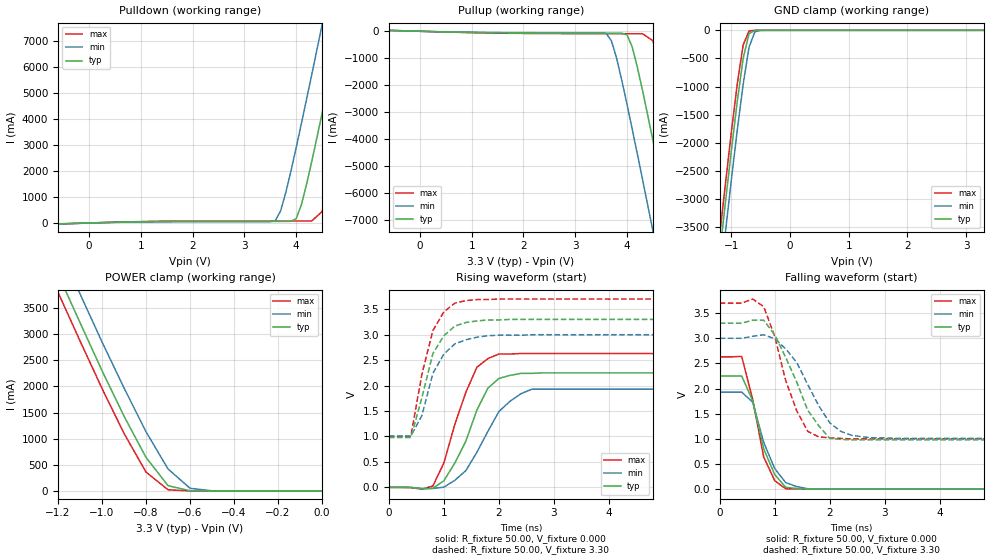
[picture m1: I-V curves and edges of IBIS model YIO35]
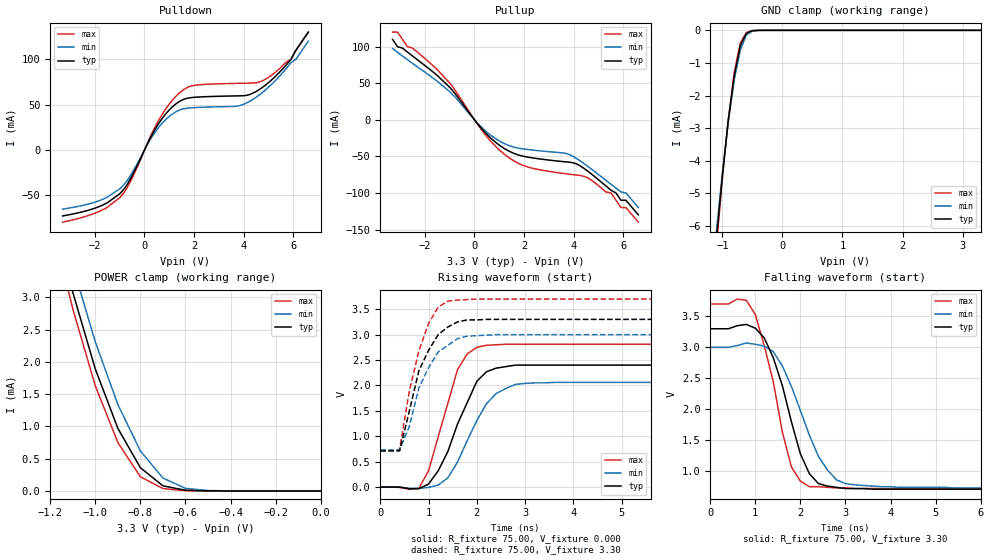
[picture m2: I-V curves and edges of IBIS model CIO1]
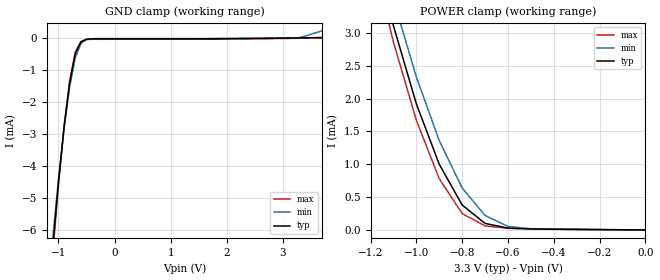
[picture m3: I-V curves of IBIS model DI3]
|   * 9e4101a.ibs * IBIS 2.1 Model file
| Components:
| ICS9e4101a   CK410 CLOCK
| Rev History
| Rev No.   Description
| 1.0   Initial release with Updated Parasitic Parameters
[IBIS Ver]   2.1
[Comment char]  |_char
[File name]   9e4101a.ibs
[Date]   Jan. 27, 2004
[File Rev]   1.0
[Source]   Originated at Integrated Circuit Systems, Inc.
[Disclaimer] (C) Copyright Integrated Circuit Systems, Inc. 2002
   All rights reserved
ICS hereby grants the user of this IBIS model a non-exclusive,
nontransferable license to use this IBIS model under the following terms.
Before using this IBIS model, the user should read this license.
If the user does not accept these terms,  the IBIS model should be
returned to ICS within 30 days.
   The user is granted this license only to use the IBIS model and
is not granted rights to sell, load, rent, lease or license the IBIS
model in whole or in part, or in modified form to anyone other than
user. User may modify the IBIS model to suit its specific
applications but rights to derivative works and such modifications
shall belong to ICS.
   This IBIS model is provided on an "AS IS" basis and ICS makes
absolutely no warranty with respect to the information contained
herein. ICS DISCLAIMS AND CUSTOMER WAIVES ALL WARRANTIES, EXPRESS
OR IMPLIED, INCLUDING WARRANTIES OF MERCHANTABILITY OR FITNESS FOR
A PARTICULAR PURPOSE. The entire risk as to quality and performance
is with the Customer. ACCORDINGLY, IN NO EVENT SHALL THE COMPANY BE
LIABLE FOR ANY DAMAGES, WHETHER IN CONTRACT OR TORT,INCLUDING ANY
LOST PROFITS OR OTHER INCIDENTAL, CONSEQUENTIAL, EXEMPLARY, OR
PUNITIVE DAMAGES ARISING OUT OF THE USE OR APPLICATION OF THE IBIS
model provided in this package. Further, ICS reserves the right to
make changes without notice to any product herein to improve
reliability, function, or design. ICS does not convey any license
under patent rights or any other intellectual property rights,
including those of third parties.
   ICS is not obligated to provide maintenance or support
for the licensed IBIS model.
|   COMPONENT: ICS9e4101a
[Component]   ICS9e4101a
[Manufacturer]  ICS
[Package]
| variable   typ   min   max
R_pkg   81.1m   62.2m   100.0m
L_pkg   6.7nH   4.9nH   8.5nH
C_pkg   0.53pF  0.21pF  0.85pF
[Pin]   signal_name   model_name   R_pin   L_pin   C_pin
  1   VDDPCI   POWER
  2   GND   GND
  3   PCI_3   YO49
  4   PCI_4   YO49
  5   PCI_5   YO49
  6   GND   GND
  7   VDDPCI   POWER
  8   PCI_F0/ITP_EN   YIO35
  9   PCI_F1   YO49
 10   PCI_F2   YO49
 11   VDD48   POWER
 12   USB48   YO49
 13   GND   GND
 14   DOT_96   YH15
 15   DOT_96#   YH15
 16   FS_B   YI5
 17   VTT_PWRGD#   YI3
 18   FS_A   YI5
 19   SRC_1   YH16
 20   SRC_1#   YH16
 21   VDDSRC   POWER
 22   SRC_2   YH16
 23   SRC_2#   YH16
 24   SRC_3   YH16
 25   SRC_3#   YH16
 26   SRC_4_SATA   YH16
 27   SRC_4_SATA#   YH16
 28   VDDSRC   POWER
 29   GND   GND
 30   SRC_5#   YH16
 31   SRC_5   YH16
 32   SRC_6#   YH16
 33   SRC_6   YH16
 34   VDDSRC   POWER
 35   CPU_2_ITP#/SRC_7#   YH17
 36   CPU_2_ITP/SRC_7   YH17
 37   VDD_A   POWER
 38   GND   GND
 39   IREF   YI4
 40   CPU_1#   YH17
 41   CPU_1   YH17
 42   VDDCPU   POWER
 43   CPU_0#   YH17
 44   CPU_0   YH17
 45   GND   GND
 46   SCL   DI3
 47   SDA   DIOSDA
 48   VDDREF   POWER
 49   XTAL_OUT   DIX
 50   XTAL_IN   DIX
 51   GND   GND
 52   REF   YO39
 53   FS_C   YI5
 54   PCI_0   YO49
 55   PCI_1   YO49
 56   PCI_2   YO49
|* Either 3.3V or 2.5V
|** All model are simulated with typical corner process
[Diff Pin]   inv_pin   vdiff   tdelay_typ
14   15   NA   NA
19   20   NA   NA
22   23   NA   NA
24   25   NA   NA
26   27   NA   NA
31   30   NA   NA
33   32   NA   NA
36   35   NA   NA
41   40   NA   NA
44   43   NA   NA
| Models and submodels in the file (15): YIO35 (I/O), CIO1 (I/O), DI3 (Input), DIOSDA (I/O_open_drain), DIX (Input), YI3 (Input), YI4 (Input), YI5 (Input), YH15 (Open_source), YH16 (Open_source), YH17 (Open_source), YO32 (Open_source), YO49 (Output), YO34 (Output), YO39 (Output)
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|   Model YIO35
[Model]   YIO35
Model_type   I/O
Polarity   Non-Inverting
Enable   Active-High
Vinl =   0.80V
Vinh =   2.00V
C_comp   5.50pF   5.00pF   6.00pF
[Temperature Range]   27.00   70.00   0.000
[Voltage Range]   3.30V   3.00V   3.70V
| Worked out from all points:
|   slope of the pulldown table from 0 to 0.495 V, typ, clamps not added: 18 ohm
|   slope of the pullup table from 0 to 0.495 V, typ, clamps not added: 20.5 ohm
|   GND clamp passes 1 mA (typ) near -0.55 V on its own axis
|   POWER clamp passes 1 mA (typ) near -0.53 V on its own axis
|   rising waveform, R_fixture 50.00, V_fixture 0.000: 20-80 % time 547ps typ, 623ps min, 483ps max; typ from 0 V to 2.25 V
|   rising waveform, R_fixture 50.00, V_fixture 3.30: 20-80 % time 399ps typ, 392ps min, 356ps max; typ from 0.98 V to 3.3 V
|   falling waveform, R_fixture 50.00, V_fixture 0.000: 20-80 % time 354ps typ, 371ps min, 324ps max; typ from 2.25 V to 0 V
|   falling waveform, R_fixture 50.00, V_fixture 3.30: 20-80 % time 577ps typ, 609ps min, 450ps max; typ from 3.3 V to 0.98 V
[Pulldown]
| voltage   I(typ)   I(min)   I(max)
|  -3.30   0.000A   0.000A   0.000A
|  -3.10   0.000A   0.000A   0.000A
|  -2.90   0.000A   0.000A   0.000A
|  -2.70   0.000A   0.000A   0.000A
|  -2.50   -10.00mA   0.000A   0.000A
|  -2.30   0.000A   0.000A   0.000A
|  -2.10   -10.00mA   0.000A   0.000A
|  -1.90   0.000A   -10.00mA   0.000A
|  -1.70   -1.00mA   -1.00mA   -1.00mA
|  -1.50   -1.00mA   -1.00mA   -2.00mA
|  -1.00   -4.00mA   -4.00mA   -5.00mA
|  -0.90   -7.00mA   -5.00mA   -9.40mA
|  -0.80   -14.40mA   -8.40mA   -22.50mA
|  -0.70   -32.67mA   -17.10mA   -41.37mA
-600mV    -35.01mA   -28.6mA    -38.03mA
3.6V      62.06mA    99.79mA    76.5mA
3.7V      62.12mA    470mA      76.56mA
4V        170mA      2.9A       76.74mA
4.1V      700mA      3.82A      76.82mA
4.3V      2.36A      5.7A       77.36mA
4.5V      4.21A      7.62A      440mA
4.7V      6.12A      9.55A      2.04A
4.9V      8.05A      11.49A     3.88A
5.1V      9.99A      13.45A     5.79A
5.3V      11.94A     15.41A     7.72A
6.6V      24.78A     28.25A     20.51A
[Pullup]
| voltage   I(typ)   I(min)   I(max)
|  -3.30   0.000A   0.000A   0.000A
|  -3.10   0.000A   0.000A   0.000A
|  -2.90   0.000A   0.000A   0.000A
|  -2.70   0.000A   0.000A   0.000A
|  -2.50   0.000A   0.000A   0.000A
|  -2.30   0.000A   0.000A   0.000A
|  -2.10   10.00mA   0.000A   0.000A
|  -1.90   0.000A   0.000A   0.000A
|  -1.70   1.00mA   1.00mA   1.00mA
|  -1.50   2.00mA   1.00mA   1.00mA
|  -1.00   4.00mA   3.00mA   5.00mA
|  -0.90   6.00mA   4.00mA   8.00mA
|  -0.80   11.80mA   7.00mA   18.80mA
|  -0.70   27.70mA   13.70mA   39.15mA
-600mV    32.94mA    25.47mA    36.47mA
3.6V      -71.61mA   -83.61mA   -90.07mA
3.8V      -72.17mA   -1.01A     -90.7mA
4V        -130mA     -2.71A     -91.27mA
4.1V      -580mA     -3.63A     -91.54mA
4.3V      -2.2A      -5.5A      -92.39mA
4.5V      -4.04A     -7.41A     -350mA
4.7V      -5.94A     -9.34A     -1.9A
4.9V      -7.87A     -11.28A    -3.73A
5.1V      -9.81A     -13.24A    -5.63A
5.3V      -11.76A    -15.2A     -7.56A
6.6V      -24.57A    -28.02A    -20.33A
[GND_clamp]
| voltage   I(typ)   I(min)   I(max)
-3.3V     -24.49A    -24.99A    -24.19A
-1.2V     -3.97A     -4.5A      -3.64A
-1.1V     -3.04A     -3.57A     -2.71A
-1V       -2.13A     -2.65A     -1.8A
-900mV    -1.26A     -1.77A     -950mA
-800mV    -500mA     -960mA     -260mA
-700mV    -59.48mA   -300mA     -11.49mA
-600mV    -1.79mA    -26.13mA   -340uA
-500mV    -67.84uA   -1.03mA    -21.49uA
3.3V      57.13pA    2.39uA     37.15pA
[POWER_clamp]
| voltage   I(typ)   I(min)   I(max)
-3.3V     24.69A     25.21A     24.36A
-1.2V     4.15A      4.71A      3.8A
-1.1V     3.22A      3.77A      2.87A
-1V       2.3A       2.85A      1.96A
-900mV    1.43A      1.97A      1.1A
-800mV    640mA      1.13A      360mA
-700mV    100mA      420mA      21.62mA
-600mV    3.24mA     50.3mA     340uA
-500mV    69.94uA    2.02mA     5.17uA
0V        57.13pA    250pA      59.61pA
[Ramp]
| variable   typ   min   max
dV/dt_r   1.35/0.48n   1.16/0.59n   1.58/0.40n
dV/dt_f   1.39/0.52n   1.19/0.58n   1.62/0.38n
R_load = 50.00
[Rising Waveform]
R_fixture = 50.00
V_fixture = 0.000
V_fixture_min = 0.000
V_fixture_max = 0.000
| time   V(typ)   V(min)   V(max)
0s        0V         0V         0V
800ps     -18.14mV   -21.27mV   27.31mV
1ns       130mV      3.99mV     480mV
1.2ns     480mV      140mV      1.24V
1.4ns     910mV      330mV      1.87V
1.6ns     1.52V      690mV      2.36V
1.8ns     1.95V      1.1V       2.53V
2ns       2.14V      1.49V      2.62V
2.6ns     2.24V      1.93V      2.63V
10ns      2.25V      1.93V      2.63V
[Rising Waveform]
R_fixture = 50.00
V_fixture = 3.30
V_fixture_min = 3.00
V_fixture_max = 3.70
| time   V(typ)   V(min)   V(max)
0s        980mV      1.01V      1V
400ps     980mV      1.01V      1.01V
600ps     1.76V      1.41V      2.22V
800ps     2.63V      2.24V      3.08V
1ns       2.98V      2.62V      3.45V
1.2ns     3.17V      2.82V      3.62V
1.4ns     3.24V      2.9V       3.67V
1.6ns     3.27V      2.95V      3.69V
2ns       3.29V      2.99V      3.7V
10ns      3.3V       3V         3.7V
[Falling Waveform]
R_fixture = 50.00
V_fixture = 0.000
V_fixture_min = 0.000
V_fixture_max = 0.000
| time   V(typ)   V(min)   V(max)
0s        2.25V      1.93V      2.63V
400ps     2.25V      1.93V      2.64V
600ps     1.76V      1.73V      1.78V
800ps     800mV      930mV      640mV
1ns       290mV      410mV      170mV
1.2ns     37.2mV     130mV      7.42mV
1.4ns     13.61mV    51.13mV    4.51mV
1.6ns     1.96mV     9.67mV     2.07mV
1.8ns     1.77mV     3.5mV      1.06mV
10ns      0V         0V         -4.02uV
[Falling Waveform]
R_fixture = 50.00
V_fixture = 3.30
V_fixture_min = 3.00
V_fixture_max = 3.70
| time   V(typ)   V(min)   V(max)
0s        3.3V       3V         3.7V
600ps     3.36V      3.04V      3.78V
800ps     3.36V      3.07V      3.63V
1ns       3.07V      2.99V      3.04V
1.4ns     2.13V      2.52V      1.56V
1.6ns     1.57V      2.08V      1.15V
1.8ns     1.26V      1.66V      1.04V
2.2ns     990mV      1.15V      1.01V
2.8ns     980mV      1.02V      1V
10ns      980mV      1.01V      1V
|   Model CIO1
[Model]   CIO1
Model_type   I/O
Polarity   Non-Inverting
Enable   Active-High
Vinl =   0.80V
Vinh =   2.00V
Vmeas =   1.50V
Cref =  30.00pF
Rref =  0.000
Vref =   1.50V
C_comp   5.50pF   5.00pF   6.00pF
[Temperature Range]   27.00   70.00   0.000
[Voltage Range]   3.30V   3.00V   3.70V
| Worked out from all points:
|   slope of the pulldown table from 0 to 0.495 V, typ, clamps not added: 19.1 ohm
|   slope of the pullup table from 0 to 0.495 V, typ, clamps not added: 25.2 ohm
|   GND clamp passes 1 mA (typ) near -0.76 V on its own axis
|   POWER clamp passes 1 mA (typ) near -0.90 V on its own axis
|   rising waveform, R_fixture 75.00, V_fixture 0.000: 20-80 % time 640ps typ, 658ps min, 509ps max; typ from 0 V to 2.4 V
|   rising waveform, R_fixture 75.00, V_fixture 3.30: 20-80 % time 527ps typ, 529ps min, 456ps max; typ from 0.71 V to 3.3 V
|   falling waveform, R_fixture 75.00, V_fixture 3.30: 20-80 % time 611ps typ, 758ps min, 545ps max; typ from 3.3 V to 0.71 V
[Pulldown]
| voltage   I(typ)   I(min)   I(max)
-3.3V     -72.63mA   -65.12mA   -79.48mA
-1.9V     -63.07mA   -56.53mA   -68.55mA
-1V       -48.22mA   -42.76mA   -52.51mA
-600mV    -33.44mA   -29.63mA   -36.4mA
600mV     30.43mA    25.97mA    34.22mA
1.5V      54.98mA    44.93mA    65.01mA
2.1V      58.33mA    46.94mA    71.65mA
3.7V      59.68mA    48.27mA    73.49mA
4.5V      64.57mA    58.27mA    74.15mA
5.1V      76.76mA    71.89mA    82.02mA
5.9V      99.94mA    96.31mA    100mA
6.6V      130mA      120mA      130mA
[Pullup]
| voltage   I(typ)   I(min)   I(max)
-3.3V     110mA      97.72mA    120mA
-3.1V     100mA      92.38mA    120mA
-2.7V     92.63mA    82.25mA    100mA
-1V       44.48mA    38.53mA    50.43mA
400mV     -16.28mA   -13.82mA   -18.88mA
1.3V      -41.19mA   -33.92mA   -49.62mA
2.2V      -51.32mA   -40.82mA   -65.01mA
4.2V      -61.86mA   -54.87mA   -75.91mA
5.5V      -96.33mA   -88.16mA   -100mA
5.9V      -110mA     -98.63mA   -120mA
6.1V      -110mA     -100mA     -120mA
6.6V      -130mA     -120mA     -140mA
[GND_clamp]
| voltage   I(typ)   I(min)   I(max)
-3.3V     -62.07mA   -58.08mA   -64.92mA
-1.1V     -6.47mA    -6.2mA     -6.68mA
-1V       -4.49mA    -4.4mA     -4.57mA
-900mV    -2.76mA    -2.81mA    -2.73mA
-800mV    -1.38mA    -1.51mA    -1.28mA
-700mV    -470uA     -600uA     -390uA
-600mV    -95.19uA   -150uA     -65.17uA
-500mV    -11.85uA   -25.34uA   -6.58uA
-400mV    -1.04uA    -3.14uA    -430nA
3.3V      64.28pA    60.1nA     41.35pA
[POWER_clamp]
| voltage   I(typ)   I(min)   I(max)
-3.3V     65.33mA    62.28mA    68.22mA
-1.2V     4.48mA     4.84mA     4.26mA
-1.1V     3.08mA     3.49mA     2.82mA
-1V       1.89mA     2.31mA     1.63mA
-900mV    970uA      1.34mA     750uA
-800mV    360uA      620uA      220uA
-700mV    78.95uA    200uA      36.79uA
-600mV    10.62uA    39.86uA    3.78uA
-500mV    1.06uA     5.73uA     280nA
0V        64.28pA    210pA      60.75pA
[Ramp]
| variable   typ   min   max
dV/dt_r   1.44/0.60n   1.24/0.65n   1.69/0.44n
dV/dt_f   1.56/0.60n   1.36/0.73n   1.79/0.47n
R_load = 75.00
[Rising Waveform]
R_fixture = 75.00
V_fixture = 0.000
V_fixture_min = 0.000
V_fixture_max = 0.000
| time   V(typ)   V(min)   V(max)
0s        0V         96.23uV    190uV
800ps     -32.86mV   -28.35mV   -25.18mV
1ns       58.81mV    -6.2mV     320mV
1.2ns     320mV      37.85mV    990mV
1.6ns     1.24V      490mV      2.31V
1.8ns     1.66V      910mV      2.62V
2ns       2.08V      1.31V      2.75V
2.4ns     2.34V      1.84V      2.8V
3ns       2.4V       2.04V      2.81V
10ns      2.4V       2.06V      2.81V
[Rising Waveform]
R_fixture = 75.00
V_fixture = 3.30
V_fixture_min = 3.00
V_fixture_max = 3.70
| time   V(typ)   V(min)   V(max)
0s        710mV      730mV      720mV
400ps     710mV      730mV      740mV
600ps     1.49V      1.19V      1.88V
800ps     2.29V      1.95V      2.68V
1ns       2.69V      2.35V      3.22V
1.2ns     3V         2.66V      3.54V
1.4ns     3.15V      2.79V      3.66V
1.8ns     3.29V      2.97V      3.69V
2.4ns     3.3V       3V         3.7V
10ns      3.3V       3V         3.7V
[Falling Waveform]
R_fixture = 75.00
V_fixture = 3.30
V_fixture_min = 3.00
V_fixture_max = 3.70
| time   V(typ)   V(min)   V(max)
0s        3.3V       3V         3.7V
800ps     3.37V      3.07V      3.76V
1ns       3.31V      3.05V      3.53V
1.4ns     2.83V      2.93V      2.44V
1.6ns     2.38V      2.7V       1.63V
1.8ns     1.8V       2.37V      1.07V
2.2ns     960mV      1.58V      750mV
2.6ns     760mV      1.02V      740mV
3ns       720mV      800mV      730mV
10ns      710mV      730mV      720mV
|   Model DI3
[Model]   DI3
Model_type   Input
Polarity   Inverting
Vinl =   0.80V
Vinh =   2.00V
C_comp   5.50pF   5.00pF   6.00pF
[Temperature Range]   27.00   70.00   0.000
[Voltage Range]   3.30V   3.00V   3.70V
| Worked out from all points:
|   GND clamp passes 1 mA (typ) near -0.75 V on its own axis
|   POWER clamp passes 1 mA (typ) near -0.90 V on its own axis
[GND_clamp]
| voltage   I(typ)   I(min)   I(max)
-3.3V     -62.1mA    -58.1mA    -64.96mA
-1.1V     -6.5mA     -6.22mA    -6.72mA
-1V       -4.52mA    -4.42mA    -4.61mA
-900mV    -2.79mA    -2.83mA    -2.77mA
-800mV    -1.41mA    -1.53mA    -1.33mA
-700mV    -500uA     -620uA     -440uA
-600mV    -130uA     -180uA     -110uA
-500mV    -42.15uA   -47.42uA   -49.41uA
-400mV    -31.3uA    -25.2uA    -43.22uA
3.3V      64.28pA    7.06uA     -12.09uA
3.7V      11.66uA    220uA      7.53nA
[POWER_clamp]
| voltage   I(typ)   I(min)   I(max)
-3.3V     65.46mA    62.39mA    68.37mA
-1.2V     4.51mA     4.87mA     4.31mA
-1.1V     3.11mA     3.51mA     2.86mA
-1V       1.92mA     2.33mA     1.67mA
-900mV    1mA        1.36mA     780uA
-800mV    380uA      640uA      250uA
-700mV    100uA      220uA      61.82uA
-600mV    28.45uA    54.53uA    25.09uA
-500mV    15.73uA    17.8uA     17.86uA
0V        64.28pA    2.84nA     7.53nA
